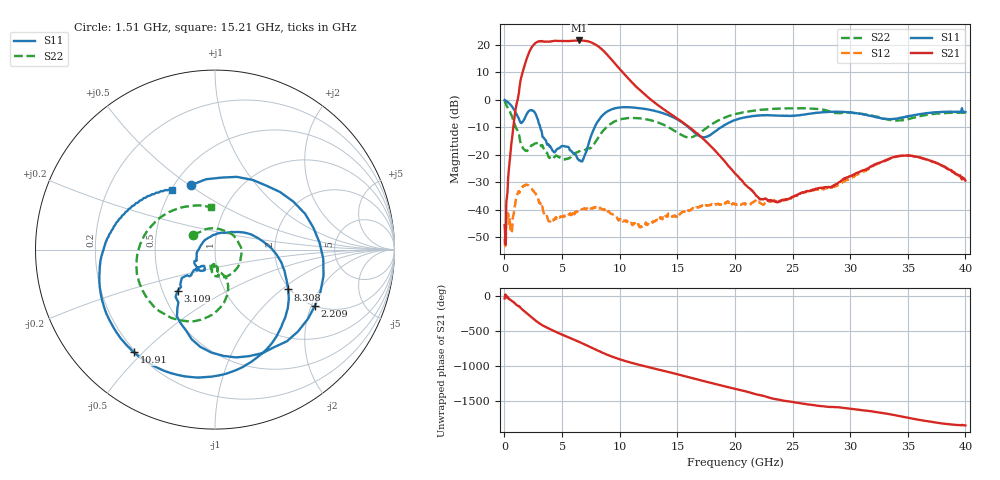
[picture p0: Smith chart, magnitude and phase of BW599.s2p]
!Agilent Technologies,N5244A,MY49441013,A.09.90.07
!Agilent N5244A: A.09.90.07
!Date: Wednesday, May 21, 2014 11:11:09
!Correction: S11(Full 2 Port with power(1,2))
!S21(Full 2 Port with power(1,2))
!S12(Full 2 Port with power(1,2))
!S22(Full 2 Port with power(1,2))
!S2P File: Measurements: S11, S21, S12, S22:
# Hz S  dB  R 50
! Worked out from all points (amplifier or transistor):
!   801 points, 10 MHz to 40 GHz, reference 50 ohm
!   highest |S21| = 21.6 dB at 6.458 GHz (marker M1)
!   |S21| within 3 dB of that: 2.29 GHz to 8.391 GHz (6.101 GHz wide, 114 % of centre)
!   unconditionally stable (mu >= 1): start of sweep to end of sweep
!   at 6.658 GHz: K = 4.14, MAG = 21.7 dB, |S12| = -40.0 dB
!   at 20 GHz: K = 506.74, MAG = -24.4 dB, |S12| = -38.2 dB
!   at 40 GHz: K = 187.22, MAG = -25.7 dB, |S12| = -29.4 dB
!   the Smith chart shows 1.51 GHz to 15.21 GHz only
!   S11 on the Smith chart (normalised r, x): 1.51 GHz: 0.60, +0.51; 2.209 GHz: 1.99, -2.12; 3.109 GHz: 0.60, -0.30; 8.308 GHz: 1.96, -1.11; 10.91 GHz: 0.19, -0.47; 15.21 GHz: 0.50, +0.41
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1e7  -0.06 -1.8  -45.70 -31.2  -50.67 38.7  -0.15 -3.6
1.509625e9  -8.33 110.6  9.01 176.3  -31.88 -19.8  -16.86 146.6
1.859538e9  -5.82 31.6  14.15 126.9  -30.93 -65.6  -18.61 85.2
2.20945e9  -3.89 -29.6  17.95 77.9  -31.73 -112.5  -17.39 20.2
2.709325e9  -5.22 -98.5  20.75 10.9  -34.17 -173.0  -15.87 -43.0
3.109225e9  -10.23 -132.3  21.32 -36.2  -37.66 141.1  -16.08 -79.1
3.459138e9  -14.26 -132.8  21.13 -69.4  -41.65 109.6  -18.55 -99.0
3.859038e9  -16.45 -134.2  21.16 -102.4  -44.24 89.0  -21.07 -102.3
4.758812e9  -17.64 -118.1  21.41 -172.0  -42.80 29.3  -21.03 -98.5
5.708575e9  -18.45 -148.7  21.44 121.5  -41.29 -28.9  -21.10 -84.8
6.458388e9  -22.07 155.5  21.60 68.0  -40.71 -60.7  -18.81 -83.7
6.708325e9  -22.43 118.8  21.55 49.7  -39.94 -73.5  -18.51 -84.0
7.40815e9  -14.45 30.1  21.09 -4.3  -39.40 -105.4  -17.70 -78.5
8.307925e9  -6.67 -28.6  18.90 -73.9  -39.38 -149.1  -12.67 -71.5
9.257688e9  -3.56 -74.4  14.79 -139.8  -41.57 174.2  -8.66 -94.2
1.090728e10  -2.74 -128.3  6.98 132.2  -45.06 137.6  -6.65 -138.6
1.335666e10  -4.39 174.1  -2.10 30.0  -43.29 112.0  -8.34 161.5
1.52062e10  -7.70 125.7  -7.46 -45.6  -41.66 76.2  -12.46 95.2
2.0005e10  -7.41 -100.4  -26.80 114.9  -38.16 -40.3  -5.23 -101.6
2.670332e10  -4.95 178.8  -32.90 -118.5  -33.19 -137.3  -3.24 165.7
3.335166e10  -7.05 115.6  -21.59 112.2  -21.67 110.9  -7.35 107.9
4e10  -4.47 51.3  -29.43 -51.8  -29.44 -48.2  -4.72 51.4
